
DATA_BLOCK DB3499
TITLE=
VERSION : 0.1

STRUCT
   CM_ID : STRING  [8 ] := '=PRM'; //COMPOSITE MACHINE
   STATION_ID : STRING  [8 ] := '++OP10'; //STATION - TRATTO - ZONE
   ELEMENT_ID : STRING  [8 ] := '+82PP40'; //ELEMENT
   DB_ID : INT := 0 ; //DB SIZE OR TYPE
   PART_STYLE : STRING  [12 ]; //PART STYLE ON LAST STATION
   ACT_CYCLE_TIME : INT ; //ACTUAL CYCLE TIME FOR THIS STYLE
   COUNT_GOOD : INT ; //COUNTER GOOD PIECES
   COUNT_SCRAP : INT ; //COUNTER SCRAP PIECES
   SPARE_00 : ARRAY  [0 .. 15 ] OF //SPARE INTEGER
   INT ;
   SPARE_01 : ARRAY  [0 .. 17 ] OF //SPARE INTEGER
   INT ;
   CODE_EVENT : ARRAY  [0 .. 7 ] OF //CODE EVENT - EXTENDED FAULT CODE DIAGNOSTIC
   INT ;
   EVENT : STRUCT
E0000 : BOOL ; //+82PP40-U1;MS.GENERALI ERRORE;1
E0001 : BOOL ; //+82PP40-U1;MS.GENERALI AVVERTIMENTO;2
E0002 : BOOL ; //+82PP40-U1;MS.MODALITA MANUALE;16
E0003 : BOOL ; //+82PP40-U1;MS.MODO AUTOMATICO;19
E0004 : BOOL ; //+82PP40-U1;MS.RILASCIO;17
E0005 : BOOL ; //+82PP40-U1; MS. MOTORE ON;58
E0006 : BOOL ; //+82PP40-U1; MS. MOTORE OFF;58
E0007 : BOOL ; //+82PP40-U1; MS. MOTORE ON FRONTE POSITIVO;58
E0008 : BOOL ; //+82PP40-U1; MS. FREQUENZA OK;58
E0009 : BOOL ; //+82PP40-U1; MS. LOCALE DI CONTROLLO INTERRUTTORE ABILITATO;58
E0010 : BOOL ; //+82PP40-U1; MS. ARRESTO A SUO AGIO;58
E0011 : BOOL ; //+82PP40-U1; MS. LAST TASTO PREMUTO;58
E0012 : BOOL ; //+82PP40-U1; MS. MS_14;58
E0013 : BOOL ; //+82PP40-U1; MS. MS_15;58
E0014 : BOOL ; //+82PP40-U1; MS. RES_WO_SAFETY_TEST;58
E0015 : BOOL ; //+82PP40-U1; MS. MOTORE OFF FRONTE NEGATIVO;58
E0016 : BOOL ; //+82PP40-U1;ME.MOTORE PROTEZIONE NON OK;1
E0017 : BOOL ; //+82PP40-U1;ME.RUNTIME;1
E0018 : BOOL ; //+82PP40-U1;ME.FREQUENZA CONVERTITORE PRONTO ERRORE;1
E0019 : BOOL ; //+82PP40-U1;ME.FREQUENZA CONVERTITORE INTERNO ERRORE;1
E0020 : BOOL ; //+82PP40-U1;ME.FREQUENZA CONVERTITORE DI VELOCITA ERRORE;1
E0021 : BOOL ; //+82PP40-U1;ME.FREQUENZA CONVERTITORE MOTORE SOVRACCARICO;1
E0022 : BOOL ; //+82PP40-U1; ME. FREQUENZA CONVERTITORE MOTORE SOVRACCARICO;58
E0023 : BOOL ; //+82PP40-U1;ME.FREQUENZA CONVERTITORE AVVERTIMENTO;2
E0024 : BOOL ; //+82PP40-U1; ME. FREQUENZA CONVERTITORE CORRENTE LIMITE DI ATTENZIONE;58
E0025 : BOOL ; //+82PP40-U1;ME.PTC AVVERTIMENTO;2
E0026 : BOOL ; //+82PP40-U1;ME.INTERRUTTORE PER MANUTENZIONE ERROR RILASCIO;1
E0027 : BOOL ; //+82PP40-U1;ME.INTERRUTTORE PER MANUTENZIONE ERROR CORRENTE TAGLIARE;1
E0028 : BOOL ; //+82PP40-U1; ME. ME_14;58
E0029 : BOOL ; //+82PP40-U1; ME. ME_15;58
E0030 : BOOL ; //+82PP40-U1; ME. ME_16;58
E0031 : BOOL ; //+82PP40-U1; ME. ME_17;58
E0032 : BOOL ;
E0033 : BOOL ;
E0034 : BOOL ;
E0035 : BOOL ;
E0036 : BOOL ;
E0037 : BOOL ;
E0038 : BOOL ;
E0039 : BOOL ;
E0040 : BOOL ;
E0041 : BOOL ;
E0042 : BOOL ;
E0043 : BOOL ;
E0044 : BOOL ;
E0045 : BOOL ;
E0046 : BOOL ;
E0047 : BOOL ;
E0048 : BOOL ;
E0049 : BOOL ;
E0050 : BOOL ;
E0051 : BOOL ;
E0052 : BOOL ;
E0053 : BOOL ;
E0054 : BOOL ;
E0055 : BOOL ;
E0056 : BOOL ;
E0057 : BOOL ;
E0058 : BOOL ;
E0059 : BOOL ;
E0060 : BOOL ;
E0061 : BOOL ;
E0062 : BOOL ;
E0063 : BOOL ;
END_STRUCT;
END_STRUCT;
BEGIN
CM_ID := '=PRM';
STATION_ID := '++OP10';
ELEMENT_ID := '+82PP40';
DB_ID := 0 ;
PART_STYLE := '';
ACT_CYCLE_TIME := 0;
COUNT_GOOD := 0;
COUNT_SCRAP := 0;
SPARE_00[0] := 0;
SPARE_00[1] := 0;
SPARE_00[2] := 0;
SPARE_00[3] := 0;
SPARE_00[4] := 0;
SPARE_00[5] := 0;
SPARE_00[6] := 0;
SPARE_00[7] := 0;
SPARE_00[8] := 0;
SPARE_00[9] := 0;
SPARE_00[10] := 0;
SPARE_00[11] := 0;
SPARE_00[12] := 0;
SPARE_00[13] := 0;
SPARE_00[14] := 0;
SPARE_00[15] := 0;
SPARE_01[0] := 0;
SPARE_01[1] := 0;
SPARE_01[2] := 0;
SPARE_01[3] := 0;
SPARE_01[4] := 0;
SPARE_01[5] := 0;
SPARE_01[6] := 0;
SPARE_01[7] := 0;
SPARE_01[8] := 0;
SPARE_01[9] := 0;
SPARE_01[10] := 0;
SPARE_01[11] := 0;
SPARE_01[12] := 0;
SPARE_01[13] := 0;
SPARE_01[14] := 0;
SPARE_01[15] := 0;
SPARE_01[16] := 0;
SPARE_01[17] := 0;
CODE_EVENT[0] := 0;
CODE_EVENT[1] := 0;
CODE_EVENT[2] := 0;
CODE_EVENT[3] := 0;
CODE_EVENT[4] := 0;
CODE_EVENT[5] := 0;
CODE_EVENT[6] := 0;
CODE_EVENT[7] := 0;
EVENT.E0000 := FALSE;
EVENT.E0001 := FALSE;
EVENT.E0002 := FALSE;
EVENT.E0003 := FALSE;
EVENT.E0004 := FALSE;
EVENT.E0005 := FALSE;
EVENT.E0006 := FALSE;
EVENT.E0007 := FALSE;
EVENT.E0008 := FALSE;
EVENT.E0009 := FALSE;
EVENT.E0010 := FALSE;
EVENT.E0011 := FALSE;
EVENT.E0012 := FALSE;
EVENT.E0013 := FALSE;
EVENT.E0014 := FALSE;
EVENT.E0015 := FALSE;
EVENT.E0016 := FALSE;
EVENT.E0017 := FALSE;
EVENT.E0018 := FALSE;
EVENT.E0019 := FALSE;
EVENT.E0020 := FALSE;
EVENT.E0021 := FALSE;
EVENT.E0022 := FALSE;
EVENT.E0023 := FALSE;
EVENT.E0024 := FALSE;
EVENT.E0025 := FALSE;
EVENT.E0026 := FALSE;
EVENT.E0027 := FALSE;
EVENT.E0028 := FALSE;
EVENT.E0029 := FALSE;
EVENT.E0030 := FALSE;
EVENT.E0031 := FALSE;
EVENT.E0032 := FALSE;
EVENT.E0033 := FALSE;
EVENT.E0034 := FALSE;
EVENT.E0035 := FALSE;
EVENT.E0036 := FALSE;
EVENT.E0037 := FALSE;
EVENT.E0038 := FALSE;
EVENT.E0039 := FALSE;
EVENT.E0040 := FALSE;
EVENT.E0041 := FALSE;
EVENT.E0042 := FALSE;
EVENT.E0043 := FALSE;
EVENT.E0044 := FALSE;
EVENT.E0045 := FALSE;
EVENT.E0046 := FALSE;
EVENT.E0047 := FALSE;
EVENT.E0048 := FALSE;
EVENT.E0049 := FALSE;
EVENT.E0050 := FALSE;
EVENT.E0051 := FALSE;
EVENT.E0052 := FALSE;
EVENT.E0053 := FALSE;
EVENT.E0054 := FALSE;
EVENT.E0055 := FALSE;
EVENT.E0056 := FALSE;
EVENT.E0057 := FALSE;
EVENT.E0058 := FALSE;
EVENT.E0059 := FALSE;
EVENT.E0060 := FALSE;
EVENT.E0061 := FALSE;
EVENT.E0062 := FALSE;
EVENT.E0063 := FALSE;
END_DATA_BLOCK
